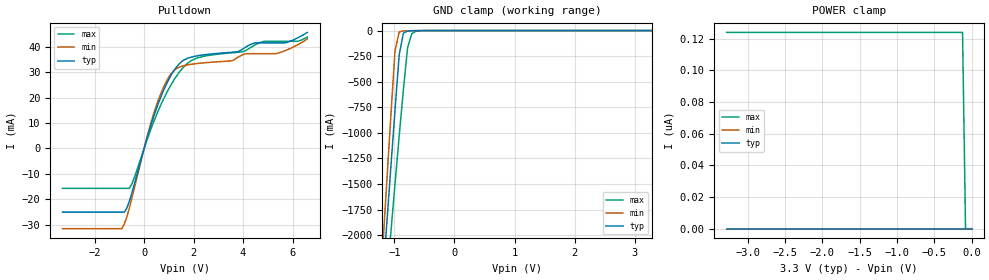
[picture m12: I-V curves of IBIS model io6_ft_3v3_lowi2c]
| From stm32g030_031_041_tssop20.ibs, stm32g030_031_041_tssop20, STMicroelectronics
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[Model]  io6_ft_3v3_lowi2c
Model_type I/O_open_drain
Polarity   Non-Inverting
Enable   Active-Low
Vinl =   0.990000V
Vinh =   2.310000V
Vmeas =  1.650000V
Cref =   30.000000pF
Rref =   500
Vref =   3.0V
C_comp   1.290400pF   1.272500pF   1.305600pF
[Temperature Range]   25.000000   -40.000000   0.125000k
[Pullup Reference]   3.300000V   3.000000V   3.600000V
[Pulldown Reference]   0.0V   0.0V   0.0V
[POWER Clamp Reference]   3.300000V   3.000000V   3.600000V
[GND Clamp Reference]   0.0V   0.0V   0.0V
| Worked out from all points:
|   slope of the pulldown table from 0 to 0.495 V, typ, clamps not added: 31.8 ohm
|   GND clamp passes 1 mA (typ) near -0.65 V on its own axis
[Pulldown]
|Voltage   I(typ)   I(min)   I(max)
-3.3V     -25.03mA   -31.54mA   -15.7mA
-900mV    -25.03mA   -31.54mA   -15.7mA
-700mV    -23.48mA   -26.96mA   -15.7mA
-500mV    -17.69mA   -19.75mA   -14.07mA
100mV     3.479mA    3.853mA    2.862mA
500mV     15.71mA    16.96mA    13.17mA
900mV     25.22mA    26.33mA    21.66mA
1.3V      31.91mA    31.32mA    28.29mA
2.2V      36.48mA    33.43mA    35.69mA
4.1V      39.78mA    37.21mA    38.43mA
5.4V      41.49mA    37.39mA    42.11mA
6.6V      45.6mA     43.04mA    43.74mA
[GND_clamp]
|Voltage   I(typ)   I(min)   I(max)
-3.3V     -9.61A     -9.635A    -9.699A
-1.2V     -2.493A    -2.184A    -2.958A
-1.13V    -1.917A    -1.512A    -2.469A
-1.06V    -1.345A    -845.6mA   -1.983A
-990mV    -779.8mA   -200.2mA   -1.503A
-920mV    -235.5mA   -14.18mA   -1.03A
-850mV    -26.06mA   -3.338mA   -574.2mA
-780mV    -4.499mA   -1.808mA   -166.4mA
-710mV    -1.722mA   -869.6uA   -29.45mA
-640mV    -806.7uA   -283.7uA   -6.281mA
3.28V     0A         0A         0A
[POWER_clamp]
|Voltage   I(typ)   I(min)   I(max)
-3.28V    0A         0A         124nA
-120mV    0A         0A         124nA
-80mV     0A         0A         0A
0V        0A         0A         0A
[Ramp]
| variable   typ   min   max
dV/dt_r  1.07520/45.58183n   0.96354/40.29803n   1.030/56.81799n
dV/dt_f  1.03164/40.73684n   0.95298/40.26549n   1.02432/43.49873n
R_load = 50.000000
